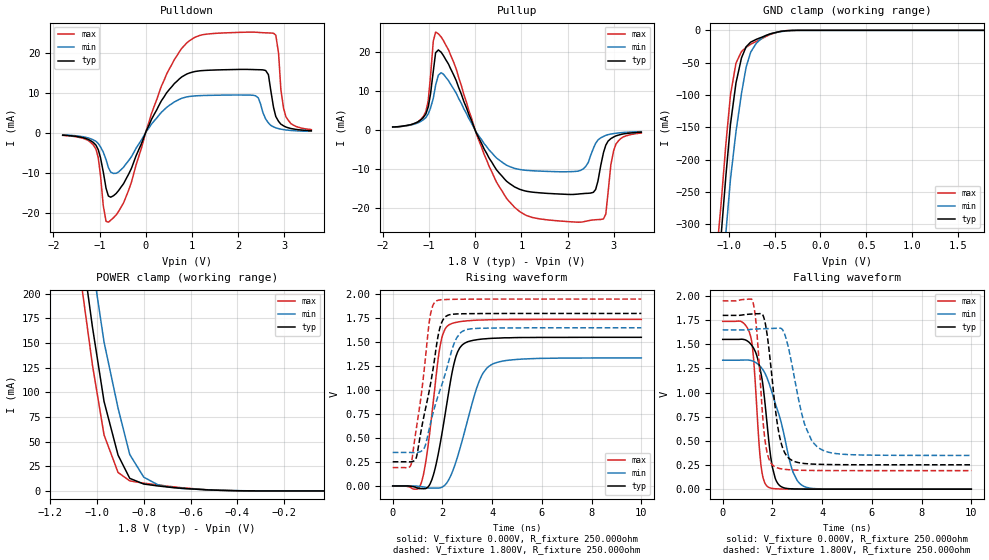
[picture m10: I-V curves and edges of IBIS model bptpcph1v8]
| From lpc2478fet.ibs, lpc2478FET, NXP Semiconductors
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| bptpcph1v8
|   Output
|   CMOS
|   Characterized at Core 1.8V and I/O 1.8V
[Model]   bptpcph1v8
Model_type   Output
Polarity   Non-Inverting
| AC Test Load Conditions
Vref   = 0
Cref   = 1.2e-11
Rref   = 1000000000
Vmeas   = 0.9
| [Process Range]   typical   min   max
| C_comp edge width   400.000ps   400.000ps   400.000ps
| C_comp Tstrobe   40.000fs   40.000fs   40.000fs
C_comp   3.039pF   2.826pF   3.273pF
[Temperature Range]   25   125   -40
[Voltage Range]   1.80V   1.65V   1.95V
[GND Clamp Reference]   0.00V   0.00V   0.00V
[Pulldown Reference]   0.00V   0.00V   0.00V
[POWER Clamp Reference]   1.80V   1.65V   1.95V
[Pullup Reference]   1.80V   1.65V   1.95V
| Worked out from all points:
|   slope of the pulldown table from 0 to 0.27 V, typ, clamps not added: 42.6 ohm
|   slope of the pullup table from 0 to 0.27 V, typ, clamps not added: 42 ohm
|   GND clamp passes 1 mA (typ) near -0.39 V on its own axis
|   POWER clamp passes 1 mA (typ) near -0.52 V on its own axis
|   rising waveform, V_fixture 0.000V, R_fixture 250.000ohm: 20-80 % time 621ps typ, 881ps min, 479ps max; typ from 0 V to 1.55 V
|   falling waveform, V_fixture 0.000V, R_fixture 250.000ohm: 20-80 % time 439ps typ, 819ps min, 273ps max; typ from 1.55 V to 0 V
|   rising waveform, V_fixture 1.800V, R_fixture 250.000ohm: 20-80 % time 643ps typ, 867ps min, 502ps max; typ from 0.252 V to 1.8 V
|   falling waveform, V_fixture 1.800V, R_fixture 250.000ohm: 20-80 % time 432ps typ, 689ps min, 301ps max; typ from 1.8 V to 0.252 V
[GND Clamp]
| ref voltage   0.00V   0.00V   0.00V
|   Voltage   I(typ)   I(min)   I(max)
-1.8V     -1.649A    -1.719A    -1.613A
-1.14V    -408mA     -495mA     -359.6mA
-1.08V    -314mA     -402mA     -264.4mA
-1.03V    -225mA     -313.1mA   -175.7mA
-980mV    -145.1mA   -230.2mA   -99.81mA
-920mV    -81.35mA   -156.7mA   -50.75mA
-860mV    -42.61mA   -97.59mA   -32.76mA
-810mV    -25.57mA   -57.29mA   -26.25mA
-760mV    -18.24mA   -33.82mA   -21.5mA
-590mV    -7.746mA   -7.76mA    -9.284mA
-370mV    -619.7uA   -1.003mA   -443.1uA
1.78V     2.377nA    739nA      118.5pA
[Power Clamp]   | Vtable = Vcc - Vpad
| ref voltage   1.80V   1.65V   1.95V
|   Voltage   I(typ)   I(min)   I(max)
-1.79V    1.607A     1.652A     1.582A
-1.07V    254mA      317.7mA    215.6mA
-1.02V    166.7mA    230.5mA    128.2mA
-970mV    90.67mA    150.9mA    56.7mA
-910mV    36.28mA    83.84mA    18.7mA
-860mV    12.75mA    36.91mA    10.18mA
-800mV    6.976mA    13.91mA    7.842mA
-740mV    5.053mA    6.276mA    6.129mA
-690mV    3.769mA    3.749mA    4.606mA
-640mV    2.697mA    2.552mA    3.27mA
-410mV    243.9uA    359.8uA    210.8uA
-30mV     2.879nA    104.9nA    138.4pA
[Pulldown]
| ref voltage   0.00V   0.00V   0.00V
|   Voltage   I(typ)   I(min)   I(max)
-1.8V     -592.6uA   -506.2uA   -645.9uA
-1.08V    -3.067mA   -2.122mA   -4.061mA
-810mV    -15.75mA   -8.653mA   -22.28mA
-480mV    -12.67mA   -8.569mA   -17.45mA
340mV     7.991mA    5.118mA    11.63mA
780mV     13.92mA    8.593mA    21.04mA
2.21V     15.79mA    9.401mA    25.09mA
2.66V     14.48mA    2.459mA    24.89mA
2.82V     4.05mA     1.224mA    24.33mA
2.93V     2.149mA    898.2uA    10.74mA
3.04V     1.427mA    704.8uA    3.976mA
3.59V     539.8uA    384.5uA    786.9uA
[Pullup]   | Vtable = Vcc - Vpad
| ref voltage   1.80V   1.65V   1.95V
|   Voltage   I(typ)   I(min)   I(max)
-1.79V    807.8uA    733.3uA    820.8uA
-1.07V    4.19mA     3.22mA     4.8mA
-860mV    19.87mA    11.53mA    25.18mA
-690mV    19.13mA    14.35mA    22.98mA
460mV     -10.2mA    -7.158mA   -13.36mA
1.12V     -15.74mA   -10.36mA   -22mA
2.28V     -16.37mA   -10.35mA   -23.66mA
2.56V     -15.99mA   -4.716mA   -23.09mA
2.78V     -5.772mA   -1.624mA   -22.82mA
2.94V     -2.188mA   -1.017mA   -8.866mA
3.05V     -1.483mA   -806.6uA   -3.589mA
3.6V      -544.3uA   -388.5uA   -762.3uA
[Ramp]
R_load   = 250.000ohm
|   dV/dt(typ)   dV/dt(min)   dV/dt(max)
dV/dt_r   431.920mV/1.075ns   287.029mV/1.255ns   583.516mV/930.000ps
dV/dt_f   423.471mV/630.000ps   256.314mV/765.000ps   625.470mV/495.000ps
[Rising Waveform]  | cubic spline decimation from 2001 points
V_fixture   = 0.000V
R_fixture   = 250.000ohm
|   Time   V(typ)   V(min)   V(max)
0s        46.48nV    2.733uV    1.511nV
1.13ns    -27.81mV   -6.104mV   17.99mV
1.35ns    -24.73mV   -16.57mV   286.2mV
1.64ns    118mV      -22.55mV   897.2mV
1.93ns    470.8mV    -17.96mV   1.49V
2.235ns   952.7mV    56.4mV     1.676V
2.73ns    1.452V     412.9mV    1.715V
3.475ns   1.529V     1.091V     1.731V
3.965ns   1.54V      1.265V     1.734V
10ns      1.551V     1.336V     1.738V
[Falling Waveform]  | cubic spline decimation from 2001 points
V_fixture   = 0.000V
R_fixture   = 250.000ohm
|   Time   V(typ)   V(min)   V(max)
0s        1.551V     1.336V     1.738V
1.115ns   1.507V     1.334V     1.59V
1.235ns   1.464V     1.324V     1.371V
1.545ns   1.191V     1.261V     237.7mV
1.845ns   521.5mV    1.11V      19.32mV
1.995ns   230.9mV    990.6mV    7.468mV
2.22ns    57.53mV    805.1mV    3.083mV
2.775ns   3.45mV     217.3mV    602.3uV
3.25ns    971.4uV    31.01mV    250.2uV
10ns      90.1nV     3.401uV    10.58nV
[Rising Waveform]  | cubic spline decimation from 2001 points
V_fixture   = 1.800V
V_fixture_min = 1.650V
V_fixture_max = 1.950V
R_fixture   = 250.000ohm
|   Time   V(typ)   V(min)   V(max)
0s        252.2mV    349.5mV    191.9mV
750ps     251.9mV    349.1mV    233.5mV
960ps     306.1mV    349.2mV    617.4mV
1.265ns   740.6mV    394mV      1.208V
1.48ns    1.008V     608.9mV    1.729V
1.735ns   1.42V      865.4mV    1.926V
2.1ns     1.761V     1.158V     1.945V
2.535ns   1.794V     1.526V     1.948V
2.9ns     1.797V     1.625V     1.949V
10ns      1.8V       1.65V      1.95V
[Falling Waveform]  | cubic spline decimation from 2001 points
V_fixture   = 1.800V
V_fixture_min = 1.650V
V_fixture_max = 1.950V
R_fixture   = 250.000ohm
|   Time   V(typ)   V(min)   V(max)
0s        1.8V       1.65V      1.95V
1.19ns    1.814V     1.656V     1.958V
1.375ns   1.817V     1.659V     1.627V
1.7ns     1.731V     1.662V     510mV
2.075ns   929.8mV    1.666V     236.1mV
2.29ns    541.9mV    1.668V     214.1mV
2.55ns    353.5mV    1.56V      204.1mV
3.28ns    266mV      685.6mV    195mV
3.875ns   257.4mV    425mV      193.1mV
10ns      252.2mV    349.5mV    191.9mV
